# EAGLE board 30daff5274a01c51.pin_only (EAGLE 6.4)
REV: C

Size 27.48 x 35.35 mm. Coordinates in mm from the lower left corner, seen from the top.
Outline: 27.48,0 9.7,0 9.7,30.48 27.48,30.48 27.48,0
Copper layers (1*16): Top 0.035mm / dielectric 1.5mm / Bottom 0.035mm
Design rules "adafruit *": minimum track width 8mil, minimum drill 15.5mil, track to track 10mil, track to pad 10mil, pad to pad 10mil, via to via 10mil, smd to smd 8mil, copper to edge 10mil, drill to drill 8mil, minimum pad ring 10mil, minimum via ring 8mil, stop-mask expansion 2mil, vias tented up to drill 20mil, thermal gap 10mil

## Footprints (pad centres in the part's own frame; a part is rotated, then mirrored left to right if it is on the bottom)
SOLDERJUMPER_ARROW_NOPASTE = smd 0.762 x 1.524: 1 -1.016,0; 2 1.016,0
0805-NO = smd 1.3 x 1.5: 1 -0.95,0; 2 0.95,0
FIDUCIAL_1MM = smd 1 x 1: 1 0,0
1X12_ROUND = drill 1 pad 1.676: 1 -13.97,0; 2 -11.43,0; 3 -8.89,0; 4 -6.35,0; 5 -3.81,0; 6 -1.27,0; 7 1.27,0; 8 3.81,0; 9 6.35,0; 10 8.89,0; 11 11.43,0; 12 13.97,0
_0805MP = smd 1.2 x 1.3: 1 -1.016,0; 2 1.016,0
SOLDERJUMPER_CLOSEDWIRE = smd 1.168 x 1.6: 1 -0.762,0; 2 0.762,0 | smd 0.635 x 0.203: WIRE 0,0
TSSOP24 = smd 0.305 x 0.991: 1 -3.575,-2.918; 2 -2.925,-2.918; 3 -2.275,-2.918; 4 -1.625,-2.918; 5 -0.975,-2.918; 6 -0.325,-2.918; 7 0.325,-2.918; 8 0.975,-2.918; 9 1.625,-2.918; 10 2.275,-2.918; 11 2.925,-2.918; 12 3.575,-2.918; 13 3.575,2.918; 14 2.925,2.918; 15 2.275,2.918; 16 1.625,2.918; 17 0.975,2.918; 18 0.325,2.918; 19 -0.325,2.918; 20 -0.975,2.918; 21 -1.625,2.918; 22 -2.275,2.918; 23 -2.925,2.918; 24 -3.575,2.918
MOUNTINGHOLE_2.5_PLATED = drill 2.5 pad 3.2: P$1 0,0

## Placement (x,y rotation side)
A0  [SOLDERJUMPER_ARROW_NOPASTE]  13.63,16.51 180 bottom
A1  [SOLDERJUMPER_ARROW_NOPASTE]  13.63,13.97 180 bottom
A2  [SOLDERJUMPER_ARROW_NOPASTE]  13.63,11.43 0 bottom
C1  10uF  [0805-NO]  17.57,21.84 270 top
FID1  FIDUCIAL""  [FIDUCIAL_1MM]  15.54,29.46 0 top
FID3  FIDUCIAL""  [FIDUCIAL_1MM]  21.89,2.54 0 top
JP1  [1X12_ROUND]  26.21,15.24 90 top
JP3  [1X12_ROUND]  10.97,15.24 270 top
R1  10K  [0805-NO]  21.51,21.84 270 top
R2  10K  [0805-NO]  19.48,21.84 90 top
R3  10K  [0805-NO]  20.49,10.29 270 top
R4  10K  [0805-NO]  18.46,10.29 90 top
R5  10K  [0805-NO]  16.56,10.29 90 top
R6  10K  [_0805MP]  15.54,21.84 90 top
SCLPU  [SOLDERJUMPER_CLOSEDWIRE]  13.76,21.59 180 bottom
SDAPU  [SOLDERJUMPER_CLOSEDWIRE]  13.76,24.13 180 bottom
U1  TCA9548APWR  [TSSOP24]  18.59,16 270 top
U$4  MOUNTINGHOLE2.5  [MOUNTINGHOLE_2.5_PLATED]  18.59,2.54 0 top
U$5  MOUNTINGHOLE2.5  [MOUNTINGHOLE_2.5_PLATED]  18.59,27.94 0 top
U$6  [PCBFEAT-REV-040]  13.89,27.18 0 bottom
U$7  [ADAFRUIT_TEXT_20MM]  24.56,20.19 270 bottom

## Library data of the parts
A0 A1 A2 FID1 FID3 U$4 U$5 = microbuilder; BOM: EXCLUDE
C1 JP1 JP3 R1-R6 SCLPU SDAPU U1 U$6 U$7 = microbuilder

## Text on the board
tPlace: VIN | SC7 | GND | SD7 | TCA9548A | SDA | SC6 | SCL | SD6 | RST | SC5 | A0 | SD5 | A1 | SC4 | A2 | SD4 | SD0 | SC3 | SC0 | I2C / Expander | SD3 | SD1 | SC2 | SC1 | SD2
bPlace: Cut to / disable / pullups | A0 | A1 | A2 | VIN: 1.8-5V

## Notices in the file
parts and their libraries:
microbuilder: This work is placed in the public domain, and may be freely used for commercial and non-commercial work with the following conditions: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
